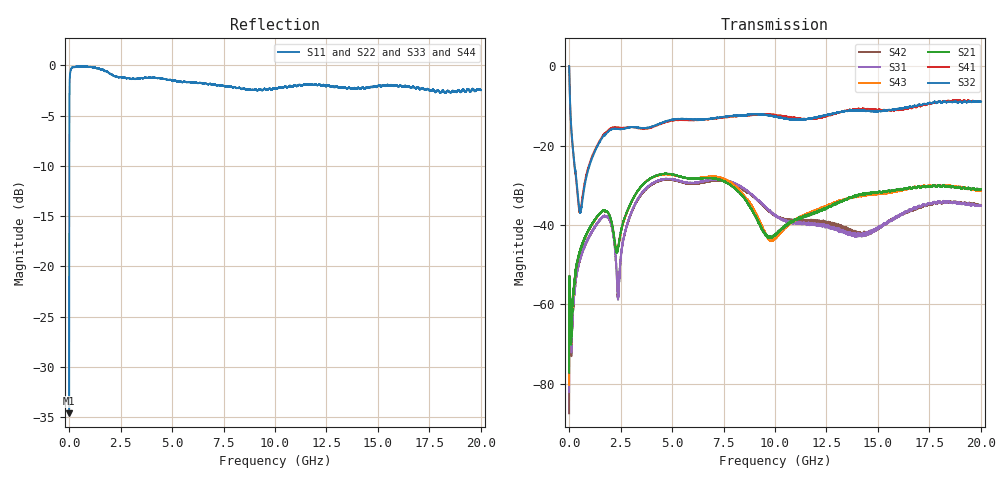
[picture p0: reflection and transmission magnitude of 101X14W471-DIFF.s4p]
!{101X14W471}
!Johanson Technology Inc.
!www.johansontechnology.com
!Test Board Conditions:
!Substrate Type  RO4350B
!Substrate Thickness  10 mil
!Substrate Dk  3.66
!TL Type: GCPW
!TL Trace Width  20 mil
!TL Gap  15 mil
!PART MODE DIFFERENTIAL
!DUT TOPOLOGY	DIFFERENTIAL 4-PORT
!Mounting Pad LxW  20x35 mil
# MHz S  dB  R 50
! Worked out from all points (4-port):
!   20001 points, 300 kHz to 20 GHz, reference 50 ohm
!   strongest paths, dB at 300 kHz, 5 GHz, 10 GHz, 15 GHz, 20 GHz:
!     S32: 0.0, -13.5, -12.7, -11.4, -8.9
!     S41: 0.0, -13.7, -12.2, -11.0, -8.9
!     S21: -77.2, -27.3, -42.5, -31.8, -31.0
!     S43: -80.3, -27.3, -43.5, -32.2, -31.3
!     S31: -82.0, -28.5, -37.5, -40.8, -35.2
!     S42: -87.4, -28.6, -37.6, -40.9, -34.9
!   lowest |S11| = -34.6 dB at 300 kHz (marker M1), VSWR 1.04, Z = 50 - j1.86 ohm
!   |S11| at or under -10 dB: start of sweep to 5.642 MHz
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0.3  -34.60 -88.1  -77.72 170.9  -83.55 16.1  -0.02 -1.2
     -77.19 68.2  -35.26 -91.3  -0.02 -1.0  -76.98 138.5
     -82.03 88.9  -0.01 -0.9  -34.74 -89.4  -74.70 39.2
     -0.02 -1.2  -87.40 113.9  -80.25 20.1  -34.69 -87.4
544.292  -0.15 176.2  -46.18 77.5  -48.41 76.5  -36.57 8.8
         -46.29 79.0  -0.24 175.1  -36.89 -1.7  -48.54 75.8
         -48.34 75.7  -36.81 -2.1  -0.16 175.2  -46.34 77.7
         -36.68 8.6  -48.39 76.1  -46.26 77.6  -0.13 174.8
1853.272  -0.63 162.1  -36.67 31.6  -37.90 21.2  -16.34 48.5
          -36.68 31.7  -0.63 161.9  -16.71 48.5  -37.98 21.6
          -37.90 21.5  -16.72 48.6  -0.57 162.5  -36.68 32.7
          -16.34 48.2  -38.02 21.6  -36.76 32.2  -0.65 163.0
2392.264  -1.18 162.2  -45.43 73.5  -58.45 57.4  -15.44 29.0
          -45.30 73.0  -1.04 161.5  -15.85 30.8  -57.71 60.8
          -57.90 57.6  -15.83 30.7  -1.03 162.4  -45.27 73.2
          -15.46 29.1  -57.39 60.4  -45.23 72.8  -1.13 163.4
4226.237  -1.26 153.8  -27.55 45.5  -29.04 40.2  -14.96 23.2
          -27.58 45.3  -1.35 154.8  -14.84 23.9  -29.15 41.2
          -29.02 40.2  -14.82 23.8  -1.26 153.4  -27.59 46.0
          -15.01 23.4  -29.18 41.5  -27.62 46.3  -1.16 154.9
9822.153  -2.41 124.3  -43.06 -20.1  -36.81 -88.5  -12.18 -11.6
          -43.27 -20.2  -2.48 120.1  -12.54 -16.4  -36.85 -81.3
          -36.96 -88.0  -12.50 -16.6  -2.46 120.8  -43.83 -25.1
          -12.21 -11.4  -36.99 -82.2  -43.85 -24.9  -2.53 125.6
20000  -2.48 67.8  -31.09 -43.7  -35.23 -87.2  -8.90 -43.1
       -31.01 -44.0  -2.80 66.3  -8.89 -47.9  -34.97 -85.2
       -35.16 -85.6  -8.89 -46.8  -2.56 64.7  -31.24 -42.4
       -8.92 -42.4  -34.94 -85.2  -31.32 -42.5  -2.60 69.7
